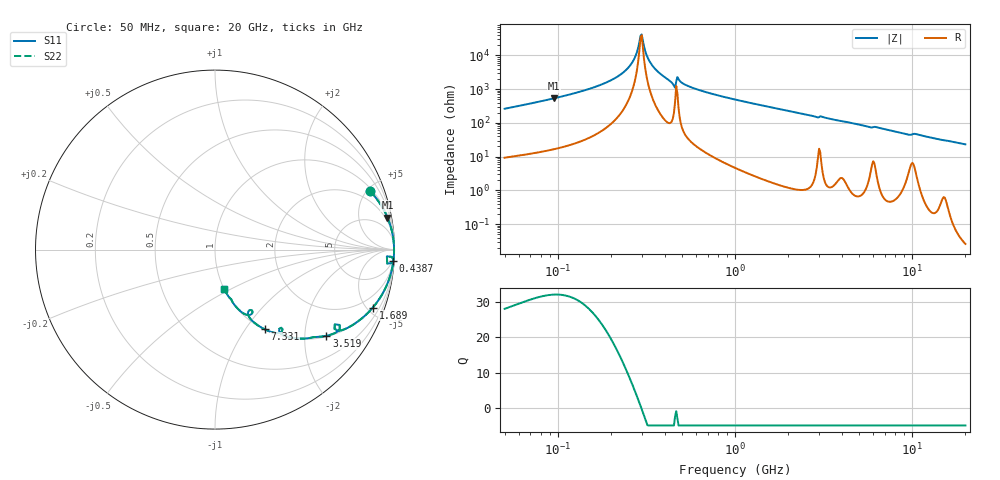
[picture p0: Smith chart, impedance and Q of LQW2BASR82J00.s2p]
!Murata Part Number: LQW2BASR82J00
!These Parameters are Measured in Series Mode Connection
!  o--[Z]--o
!Port1  Port2
!  o-------o
!Freq. Start=50[MHz] Stop=20[GHz], 401[Steps]
# Hz S RI R 50
!Freq.(Hz) S11(Real) S11(Imag) S21(Real) S21(Imag) S12(Real) S12(Imag) S22(Real) S22(Imag)
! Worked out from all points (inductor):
!   401 points, 50 MHz to 20 GHz, reference 50 ohm
!   read as one part in series: L = 804 nH near 51.52 MHz
!   highest Q = 32.2 at 95.21 MHz (marker M1), where L = 892 nH
!   self-resonance near 292.8 MHz
!   S11 on the Smith chart (normalised r, x): 50 MHz: 1.19, +5.22; 438.7 MHz: 3, -31; 1.689 GHz: 1.03, -5.44; 3.519 GHz: 1.03, -2.56; 7.331 GHz: 1.01, -1.23; 20 GHz: 1.00, -0.46
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5e7  0.8637 0.3258  0.1363 -0.3258  0.1363 -0.3258  0.8637 0.3258
9.521195e7  0.9609 0.1788  0.0391 -0.1788  0.0391 -0.1788  0.9609 0.1788
1.364002e8  0.9832 0.1128  0.0168 -0.1128  0.0168 -0.1128  0.9832 0.1128
1.925012e8  0.9936 0.0594  0.0064 -0.0594  0.0064 -0.0594  0.9936 0.0594
2.374136e8  0.9966 0.0298  0.00341 -0.0298  0.00341 -0.0298  0.9966 0.0298
2.676374e8  0.9974 0.0135  0.00256 -0.0135  0.00256 -0.0135  0.9974 0.0135
2.928045e8  0.9977 0.00127  0.0023 -0.00127  0.0023 -0.00127  0.9977 0.00127
3.017088e8  0.9977 -0.00281  0.00228 0.00281  0.00228 0.00281  0.9977 -0.00281
3.155756e8  0.9977 -0.00897  0.00233 0.00897  0.00233 0.00897  0.9977 -0.00897
3.300798e8  0.9975 -0.0152  0.00246 0.0152  0.00246 0.0152  0.9975 -0.0152
3.721004e8  0.9967 -0.0323  0.00329 0.0323  0.00329 0.0323  0.9967 -0.0323
4.387496e8  0.9916 -0.0629  0.00839 0.0629  0.00839 0.0629  0.9916 -0.0629
4.520922e8  0.9821 -0.0755  0.0179 0.0755  0.0179 0.0755  0.9821 -0.0755
4.800071e8  0.9905 -0.0498  0.00951 0.0498  0.00951 0.0498  0.9905 -0.0498
6.009314e8  0.9883 -0.0978  0.0117 0.0978  0.0117 0.0978  0.9883 -0.0978
1e9  0.9585 -0.1949  0.0415 0.1949  0.0415 0.1949  0.9585 -0.1949
1.689197e9  0.8794 -0.3228  0.1206 0.3228  0.1206 0.3228  0.8794 -0.3228
2.728004e9  0.7211 -0.4439  0.2789 0.4439  0.2789 0.4439  0.7211 -0.4439
3.519108e9  0.6207 -0.4804  0.3793 0.4804  0.3793 0.4804  0.6207 -0.4804
7.331367e9  0.2771 -0.4438  0.7229 0.4438  0.7229 0.4438  0.2771 -0.4438
7.442007e9  0.2704 -0.4404  0.7296 0.4404  0.7296 0.4404  0.2704 -0.4404
2e10  0.0509 -0.2193  0.9491 0.2193  0.9491 0.2193  0.0509 -0.2193
